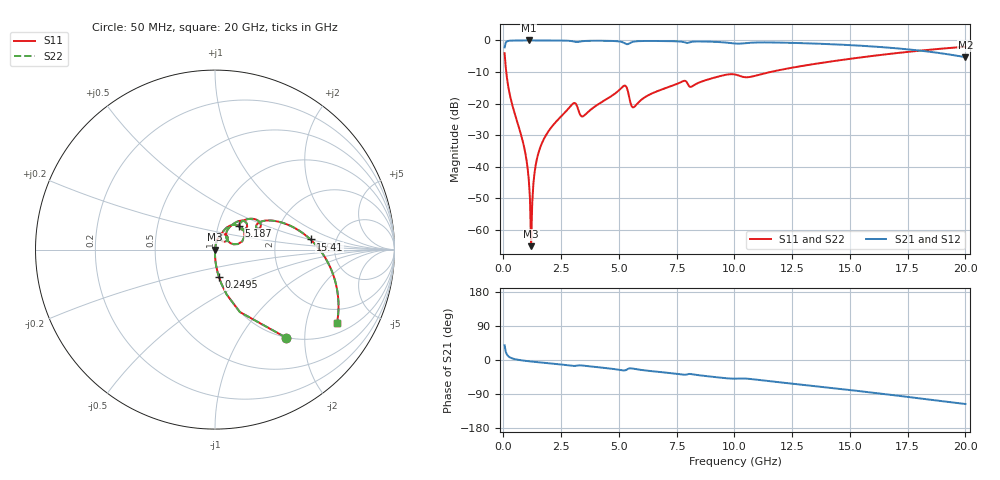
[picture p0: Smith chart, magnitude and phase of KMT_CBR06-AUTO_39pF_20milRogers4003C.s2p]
! Data measured by Modelithics Inc. support@modelithics.com 813-866-6335
! KEMET CBR06-AUTO 39pF, Pad Width= 0.851mm, Pad Length= 0.64mm, Pad Gap= 0.62mm, 20mil Rogers 4003C substrate Data, January 2022
# hz S ma R 50
! 2 Port Network Data from SP1.SP block
! freq  magS11  angS11  magS21  angS21  magS12  angS12  magS22  angS22
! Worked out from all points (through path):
!   401 points, 50 MHz to 20 GHz, reference 50 ohm
!   highest |S21| = 0.00 dB at 1.097 GHz (marker M1); lowest = -5.3 dB at 20 GHz (marker M2)
!   group delay of S21, straight-line fit = 16.2 ps
!   lowest |S11| = -65.2 dB at 1.197 GHz (marker M3), VSWR 1.00, Z = 50.1 - j0.0199 ohm
!   |S11| at or under -10 dB: 122.4 MHz to 11.56 GHz (11.44 GHz wide, 196 % of centre)
!   |S22| runs from -65.2 to -2.0 dB; largest |S21 - S12| = 0
!   S11 on the Smith chart (normalised r, x): 50 MHz: 1.00, -1.62; 249.5 MHz: 1.00, -0.31; 5.187 GHz: 1.25, +0.35; 15.41 GHz: 3.21, +0.51; 20 GHz: 1.37, -3.03
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5e7  0.6295 -51.1  0.7766 38.8  0.7766 38.8  0.6295 -51.1
2.495e8  0.1539 -81.9  0.9878 8.0  0.9878 8.0  0.1539 -81.9
8.97875e8  0.02011 -90.6  0.9993 -1.8  0.9993 -1.8  0.02011 -90.6
1.0475e9  0.009372 -90.0  0.9994 -2.9  0.9994 -2.9  0.009372 -90.0
1.097375e9  0.006175 -88.7  0.9994 -3.3  0.9994 -3.3  0.006175 -88.7
1.197125e9  0.00055 -21.2  0.9994 -4.0  0.9994 -4.0  0.00055 -21.2
1.296875e9  0.005418 79.5  0.9994 -4.6  0.9994 -4.6  0.005418 79.5
1.34675e9  0.008054 81.0  0.9994 -4.9  0.9994 -4.9  0.008054 81.0
1.4465e9  0.01313 81.8  0.9993 -5.6  0.9993 -5.6  0.01313 81.8
1.8455e9  0.03178 80.6  0.9986 -8.0  0.9986 -8.0  0.03178 80.6
2.992625e9  0.09854 60.6  0.9715 -15.4  0.9715 -15.4  0.09854 60.6
3.391625e9  0.06241 48.8  0.9702 -14.4  0.9702 -14.4  0.06241 48.8
5.187125e9  0.188 44.9  0.9268 -27.5  0.9268 -27.5  0.188 44.9
5.636e9  0.08714 39.0  0.956 -23.0  0.956 -23.0  0.08714 39.0
6.73325e9  0.1608 56.0  0.9797 -31.5  0.9797 -31.5  0.1608 56.0
7.780625e9  0.2265 44.6  0.9474 -38.6  0.9474 -38.6  0.2265 44.6
1.0025e10  0.2887 27.8  0.8942 -49.2  0.8942 -49.2  0.2887 27.8
1.06235e10  0.2623 29.1  0.9149 -49.7  0.9149 -49.7  0.2623 29.1
1.336662e10  0.4184 20.1  0.8951 -68.2  0.8951 -68.2  0.4184 20.1
1.54115e10  0.5351 6.0  0.8273 -82.1  0.8273 -82.1  0.5351 6.0
1.670825e10  0.6117 -3.7  0.7673 -91.5  0.7673 -91.5  0.6117 -3.7
2e10  0.7938 -31.0  0.5426 -116.1  0.5426 -116.1  0.7938 -31.0
